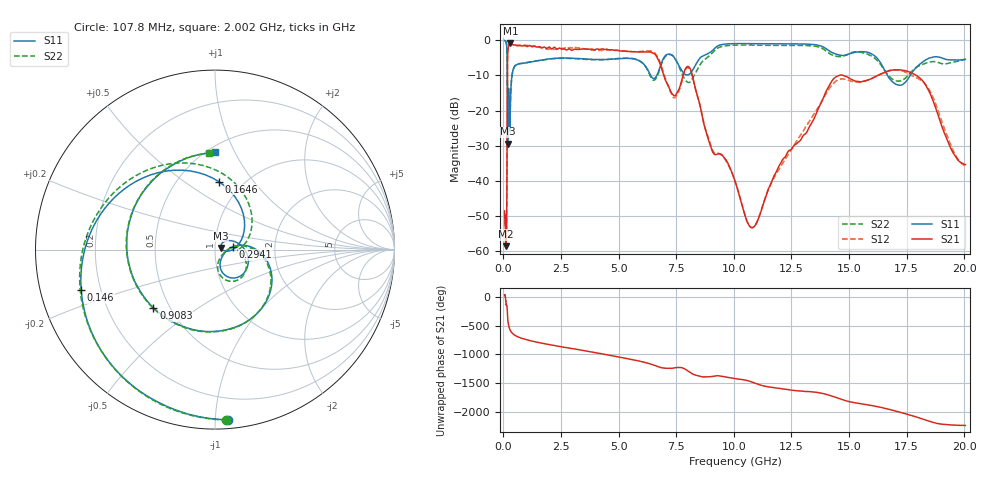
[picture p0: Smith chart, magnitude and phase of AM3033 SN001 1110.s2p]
# Hz S DB R 50
!freq MagS11 AngS11 MagS21 AngS21 MagS12 AngS12 MagS22 AngS22
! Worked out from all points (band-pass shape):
!   1601 points, 50 MHz to 20.05 GHz, reference 50 ohm
!   highest |S21| = -0.94 dB at 298.6 MHz (marker M1); lowest = -58.5 dB at 97.77 MHz (marker M2)
!   |S21| within 3 dB of the highest: 183.2 MHz to 6.567 GHz (6.384 GHz wide, 189 % of centre)
!   lowest |S11| = -29.4 dB at 181.4 MHz (marker M3), VSWR 1.07, Z = 53.4 + j0.893 ohm
!   |S11| at or under -10 dB: 166.4 MHz to 371.7 MHz (205.3 MHz wide, 76.3 % of centre); 6.385 GHz to 6.658 GHz (272.9 MHz wide, 4.18 % of centre); 16.66 GHz to 17.66 GHz (991.5 MHz wide, 5.78 % of centre)
!   |S22| runs from -26.0 to -0.1 dB; largest |S21 - S12| = 0.064
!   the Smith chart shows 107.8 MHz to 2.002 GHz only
!   S11 on the Smith chart (normalised r, x): 107.8 MHz: 0.06, -1.08; 146 MHz: 0.13, -0.15; 164.6 MHz: 0.78, +0.69; 294.1 MHz: 1.22, +0.04; 908.3 MHz: 0.41, -0.34; 2.002 GHz: 0.55, +0.84
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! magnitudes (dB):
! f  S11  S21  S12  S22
! 50 MHz  -0.1  -48.5  -50.1  -0.1
! 97.77 MHz  -0.3  -58.5  -57.6  -0.3
! 107.8 MHz  -0.4  -56.1  -56.2  -0.4
! 135.9 MHz  -1.3  -54.1  -53.8  -1.4
! 146 MHz  -2.2  -46.0  -46.0  -2.2
! 164.6 MHz  -8.4  -14.6  -14.6  -7.5
! 181.4 MHz  -29.4  -4.3  -4.2  -17.8
! 212.3 MHz  -13.9  -2.0  -2.0  -13.4
! 294.1 MHz  -19.9  -0.9  -1.0  -19.9
! 298.6 MHz  -18.6  -0.9  -1.0  -18.6
! 369.6 MHz  -10.1  -1.2  -1.1  -10.1
! 908.3 MHz  -6.5  -1.5  -1.5  -6.5
! 1.005 GHz  -6.4  -1.8  -1.5  -6.4
! 2.002 GHz  -5.3  -2.0  -2.5  -5.4
! 2.722 GHz  -5.1  -2.8  -2.4  -5.2
! 6.396 GHz  -10.1  -3.4  -3.1  -10.5
! 7.402 GHz  -4.9  -15.8  -16.4  -4.7
! 8.129 GHz  -9.3  -8.5  -8.8  -11.7
! 10.77 GHz  -1.0  -53.3  -53.3  -1.4
! 14.58 GHz  -4.2  -10.0  -11.2  -4.7
! 17.78 GHz  -8.8  -9.6  -10.2  -8.4
! 20.05 GHz  -5.5  -35.4  -35.7  -5.3
